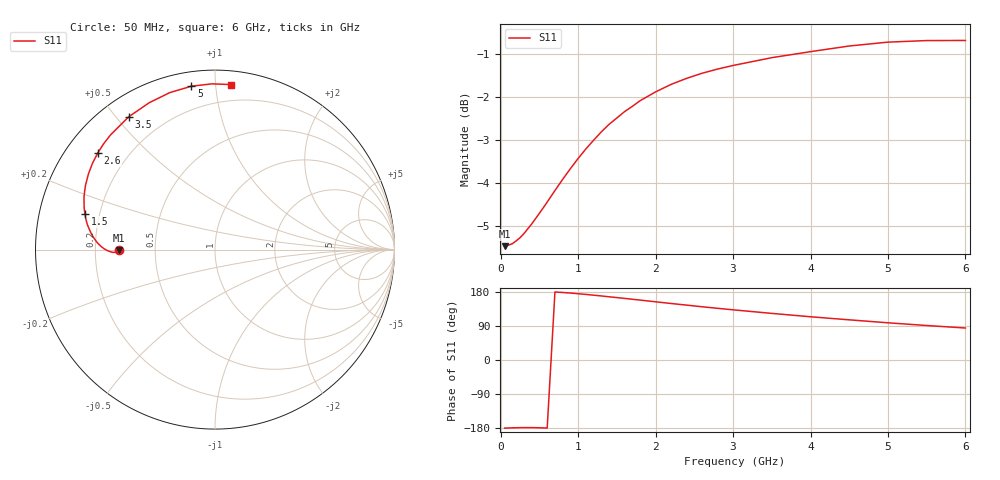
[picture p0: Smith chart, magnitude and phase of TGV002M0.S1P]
! SIEMENS Discrete & RF Semiconductors
! BAT64
! Si Schottky Diode in SOT23
! IF = 2 mA
! S-Parameters:  February  1997
# GHz  S  MA  R  50
!  f  S11
! GHz  MAG  ANG
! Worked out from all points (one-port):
!   34 points, 50 MHz to 6 GHz, reference 50 ohm
!   lowest |S11| = -5.5 dB at 50 MHz (marker M1), VSWR 3.29, Z = 15.2 - j0.119 ohm
!   |S11| at or under -10 dB: nowhere
!   S11 on the Smith chart (normalised r, x): 50 MHz: 0.30, -0.00; 1.5 GHz: 0.14, +0.13; 2.6 GHz: 0.09, +0.36; 3.5 GHz: 0.08, +0.54; 5 GHz: 0.07, +0.86; 6 GHz: 0.09, +1.10
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0.05  0.5335 -179.7
0.15  0.537 -179.0
0.2  0.5411 -178.8
0.3  0.5517 -178.5
0.4  0.5661 -178.4
0.5  0.5826 -178.8
0.6  0.6001 -179.5
0.7  0.6189 179.5
0.8  0.6377 178.2
0.9  0.6562 176.7
1.1  0.6917 173.1
1.3  0.7241 169.0
1.4  0.7387 166.8
1.5  0.7512 164.7
1.6  0.7642 162.5
1.8  0.7867 158.1
2  0.8054 153.6
2.2  0.8217 149.1
2.4  0.835 144.8
2.6  0.8465 140.5
2.8  0.856 136.4
3  0.8642 132.4
3.5  0.8824 123.0
4  0.8967 114.1
4.5  0.9104 106.0
5  0.9198 98.2
5.5  0.9237 91.0
6  0.924 84.4
